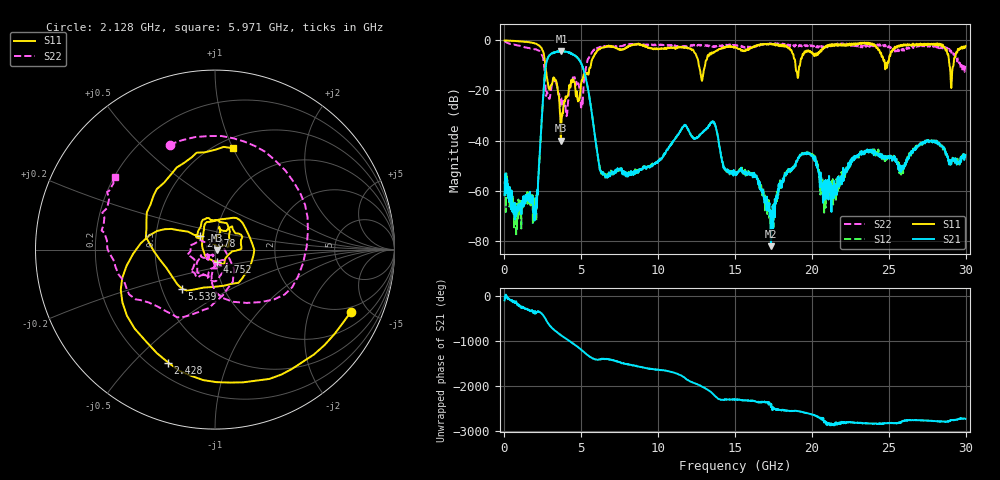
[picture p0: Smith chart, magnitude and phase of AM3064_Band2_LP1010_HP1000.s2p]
# Hz S DB R 50.0
!freq dBS11 angS11 dBS21 angS21 dBS12 angS12 dBS22 angS22
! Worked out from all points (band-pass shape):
!   1600 points, 10 MHz to 29.98 GHz, reference 50 ohm
!   highest |S21| = -4.22 dB at 3.703 GHz (marker M1); lowest = -82.2 dB at 17.33 GHz (marker M2)
!   |S21| within 3 dB of the highest: 2.811 GHz to 4.775 GHz (1.964 GHz wide, 51.8 % of centre)
!   lowest |S11| = -40.0 dB at 3.665 GHz (marker M3), VSWR 1.02, Z = 51 - j0.246 ohm
!   |S11| at or under -10 dB: 2.665 GHz to 5.616 GHz (2.951 GHz wide, 71.3 % of centre); 12.65 GHz to 13.05 GHz (403 MHz wide, 3.14 % of centre); 18.93 GHz to 19.22 GHz (285.6 MHz wide, 1.5 % of centre)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
!   |S22| runs from -30.3 to -0.3 dB; largest |S21 - S12| = 0.019
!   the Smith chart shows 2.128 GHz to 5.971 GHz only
!   S11 on the Smith chart (normalised r, x): 2.128 GHz: 1.69, -3.85; 2.428 GHz: 0.27, -0.63; 2.878 GHz: 0.84, +0.13; 4.752 GHz: 1.01, -0.14; 5.539 GHz: 0.63, -0.30; 5.971 GHz: 0.59, +1.00
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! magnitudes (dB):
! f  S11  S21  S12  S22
! 10 MHz  0.0  -61.8  -56.3  -0.3
! 741 MHz  -0.3  -70.2  -71.1  -1.9
! 2.128 GHz  -1.6  -62.1  -62.0  -3.9
! 2.428 GHz  -3.3  -31.1  -31.0  -5.8
! 2.878 GHz  -19.0  -6.4  -6.4  -22.9
! 3.665 GHz  -40.0  -4.5  -4.3  -25.1
! 3.703 GHz  -33.3  -4.2  -4.4  -23.4
! 4.752 GHz  -23.4  -6.9  -7.0  -17.3
! 5.015 GHz  -16.2  -9.6  -9.5  -24.8
! 5.539 GHz  -10.9  -23.3  -23.3  -6.0
! 5.971 GHz  -4.8  -42.1  -41.9  -3.2
! 6.608 GHz  -2.5  -54.6  -54.8  -2.3
! 10 GHz  -3.4  -48.4  -48.1  -1.9
! 13.54 GHz  -5.1  -32.6  -32.3  -2.6
! 15 GHz  -2.6  -53.4  -53.3  -1.9
! 17.33 GHz  -1.4  -82.2  -68.8  -1.4
! 19.99 GHz  -4.7  -45.8  -45.7  -2.0
! 20.89 GHz  -2.2  -55.7  -66.7  -2.8
! 25 GHz  -8.3  -46.4  -46.2  -2.3
! 28.28 GHz  -1.4  -41.2  -41.3  -3.1
! 29.08 GHz  -17.7  -48.5  -48.3  -5.1
! 29.98 GHz  -2.3  -45.8  -45.9  -10.2
